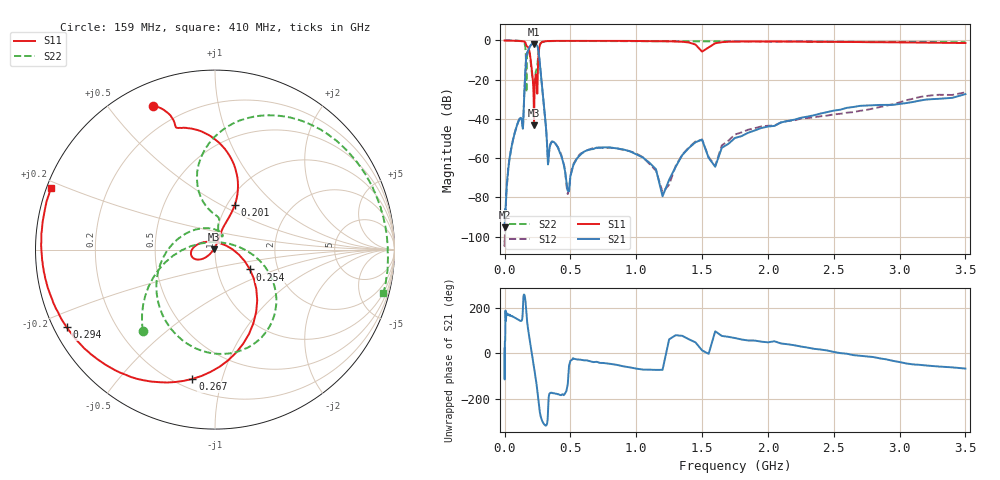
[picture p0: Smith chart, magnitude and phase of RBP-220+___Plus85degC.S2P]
! Mini-Circuits
! S2P DATA File Format
! Type: BAND PASS FILTER
! Model: RBP-220+
! All S Parameters are in dB deg format
! TEST CONDITIONS: INPUT POWER = 0 dBm @ Temperature = + 85 deg C
! 401 Frequency points
# MHz S DB R 50
!FREQ  MAG(S11)PHS(S11)MAG(S21)PHS(S21)MAG(S12)PHS(S12)MAG(S22)PHS(S22)
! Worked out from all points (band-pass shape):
!   401 points, 500 kHz to 3.5 GHz, reference 50 ohm
!   highest |S21| = -1.78 dB at 220 MHz (marker M1); lowest = -95.1 dB at 500 kHz (marker M2)
!   |S21| within 3 dB of the highest: 182.8 MHz to 256.5 MHz (73.78 MHz wide, 33.6 % of centre)
!   lowest |S11| = -43.2 dB at 224 MHz (marker M3), VSWR 1.01, Z = 49.4 + j0.239 ohm
!   |S11| at or under -10 dB: 198.9 MHz to 255.9 MHz (57.08 MHz wide, 25.1 % of centre)
!   |S22| runs from -26.4 to 0.0 dB; largest |S21 - S12| = 0.0094
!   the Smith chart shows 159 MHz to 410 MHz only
!   S11 on the Smith chart (normalised r, x): 159 MHz: 0.10, +0.66; 201 MHz: 1.08, +0.59; 254 MHz: 1.44, -0.33; 267 MHz: 0.26, -0.81; 294 MHz: 0.04, -0.25; 410 MHz: 0.01, +0.18
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0.5  -0.03 179.9  -95.11 22.3  -101.93 -157.0  -0.01 -0.1
2.5  -0.05 179.3  -89.50 52.7  -100.31 26.8  0.00 -0.7
10  -0.05 177.3  -82.37 142.5  -85.67 -161.0  0.00 -2.8
42.5  -0.10 168.8  -58.54 166.6  -58.32 166.3  -0.02 -12.7
139  -0.39 133.3  -44.96 -168.5  -45.00 -167.9  -0.47 -69.4
159  -1.19 113.2  -14.40 -132.0  -14.29 -132.8  -4.35 -131.6
166  -2.60 107.7  -7.83 176.9  -7.76 176.6  -25.92 53.1
183  -4.06 91.5  -4.74 89.3  -4.77 89.1  -4.89 -96.8
201  -11.24 66.1  -2.26 20.4  -2.24 20.1  -12.66 170.5
220  -26.75 71.9  -1.78 -48.8  -1.78 -48.9  -21.21 59.9
224  -43.17 159.6  -1.81 -63.0  -1.81 -63.0  -21.63 65.4
254  -13.00 -29.6  -3.89 170.0  -3.95 169.8  -8.65 105.3
267  -2.72 -99.9  -11.02 106.1  -11.05 107.4  -2.25 73.7
294  -0.60 -152.4  -29.41 55.2  -29.42 55.2  -0.65 32.5
327.5  -0.33 -175.4  -59.37 74.4  -59.41 76.6  -0.40 10.8
410  -0.21 159.3  -55.36 -178.7  -55.19 -178.2  -0.27 -14.5
480  -0.21 146.1  -76.54 -135.2  -78.28 -141.9  -0.25 -27.8
850  -0.23 94.4  -54.98 -50.2  -54.88 -55.3  -0.35 -74.5
1200  -0.36 45.0  -79.40 -72.2  -77.28 -37.6  -0.43 -110.4
1950  -0.55 -13.6  -44.61 51.1  -43.80 46.4  -0.56 176.6
2500  -0.75 -85.0  -35.76 6.0  -37.67 9.8  -0.64 124.0
3500  -1.30 146.6  -27.35 -66.6  -26.43 -71.8  -0.88 39.6
